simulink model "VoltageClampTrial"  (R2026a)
settings: Solver=ode1  StopTime=0.4  FixedStep=0.00001
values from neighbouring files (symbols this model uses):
  V_clamp = -0.065    [DataGeneration3.m]
libraries: LoomingNeuronLibrary x27

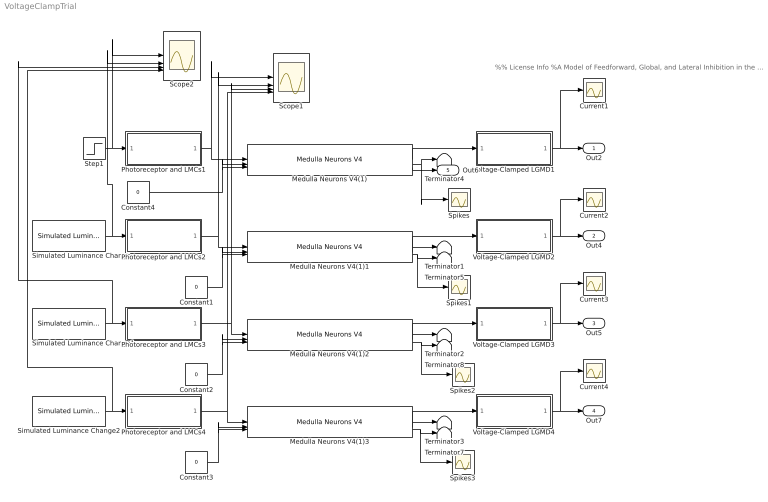
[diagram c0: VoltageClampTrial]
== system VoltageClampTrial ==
  note: %% License Info %A Model of Feedforward, Global, and Lateral Inhibition in the Locust Visual System. %This model examines the architecture and function of inhibitory mechanisms in the %visual system of locusts, namely those involved in the processing of inputs to a %key looming-sensitive neuron, the lobula giant movement detector (LGMD). %Copyright (c) 2026, Erik Olson, Travis Wiens, and Jack Gray %CITATION: %When using the model code for scientific publications, cite the following work: %Olson EGN, Wiens TK, Gray JR. A model of feedforward, global, and lateral inhibition %in the locust visual system predicts responses to looming stimuli. Biol Cybern. 2021 %Jun;115(3):245-265. doi: 10.1007/s00422-021-00876-8. Epub 2021 May 16. PMID: 33997912. %This program is free software: you can redistribute it and/or modify %it under the terms of the GNU General Public License as published by %the Free Software Foundation, either version 3 of the License, or %(at your option) any later version. %This program is distributed in the hope that it will be useful, %but WITHOUT ANY WARRANTY; without even the implied warranty of %MERCHANTABILITY or FITNESS FOR A PARTICULAR PURPOSE. See the %GNU General Public License for more details. %You should have received a copy of the GNU General Public License %along with this program. If not, see <https://www.gnu.org/licenses/>. %Contact: erik.olson@usask.ca
  Constant{1..4} (4 alike) : Constant  Value=0
  Current{1..4} (4 alike) : Scope
  Medulla Neurons V4(1){,1..3} (4 alike) : LoomingNeuronLibrary/Medulla Neurons V4  K_in_ex=K_E_m  K_in_lateral=0  K_in_global=0  g_m=g_L_m  c_m=c  E_rev_ex=E_E  E_rev_inh=E_I  E_rest=E_L  V_t=V_t  Delta_t=Delta_t_m  V_fire=V_fire  tau=tau_alpha_m  g_med_adap_inc=Delta_g_A_m  tau_med_adap=tau_A_m  E_rev_adap=E_A  g_noise=g_N_m  noise_T=T_noise  radius=1
  Photoreceptor and LMCs1 : Subsystem
  Photoreceptor and LMCs2 : Subsystem
  Photoreceptor and LMCs3 : Subsystem
  Photoreceptor and LMCs4 : Subsystem
  Scope1 : Scope  NumInputPorts=4
  Scope2 : Scope  NumInputPorts=4
  Simulated Luminance Change : LoomingNeuronLibrary/Simulated Luminance Change  duration=0.083  start=0
  Simulated Luminance Change1 : LoomingNeuronLibrary/Simulated Luminance Change  duration=0.183  start=0
  Simulated Luminance Change2 : LoomingNeuronLibrary/Simulated Luminance Change  duration=0.350  start=0
  Spikes{,1..3} (4 alike) : Scope
  Step1 : Step  Time=0.00001  InitialValue=1  FinalValue=0  SampleTime=0
  Terminator{1..5,7..8} (7 alike) : Terminator
  Voltage-Clamped LGMD1 : Subsystem
  Voltage-Clamped LGMD2 : Subsystem
  Voltage-Clamped LGMD3 : Subsystem
  Voltage-Clamped LGMD4 : Subsystem
  Out2 : Outport  VectorParamsAs1DForOutWhenUnconnected=off
  Out4 : Outport  Port=2  VectorParamsAs1DForOutWhenUnconnected=off
  Out5 : Outport  Port=3  VectorParamsAs1DForOutWhenUnconnected=off
  Out7 : Outport  Port=4  VectorParamsAs1DForOutWhenUnconnected=off
  Out6 : Outport  Port=5  VectorParamsAs1DForOutWhenUnconnected=off
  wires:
  Simulated Luminance Change/1 -> Photoreceptor and LMCs2/1(In1), Scope2/2
  Photoreceptor and LMCs4/1(Out1) -> Medulla Neurons V4(1)3/1, Scope1/4
  Medulla Neurons V4(1)2/1 -> Voltage-Clamped LGMD3/1(In1)
  Photoreceptor and LMCs2/1(Out1) -> Medulla Neurons V4(1)1/1, Scope1/2
  Simulated Luminance Change1/1 -> Photoreceptor and LMCs3/1(In1), Scope2/3
  Photoreceptor and LMCs1/1(Out1) -> Medulla Neurons V4(1)/1, Scope1/1
  Medulla Neurons V4(1)3/2 -> Terminator3/1
  Medulla Neurons V4(1)3/3 -> Spikes3/1, Terminator7/1
  Medulla Neurons V4(1)2/2 -> Terminator2/1
  Medulla Neurons V4(1)2/3 -> Spikes2/1, Terminator8/1
  Constant3/1 -> Medulla Neurons V4(1)3/3, Medulla Neurons V4(1)3/2
  Medulla Neurons V4(1)3/1 -> Voltage-Clamped LGMD4/1(In1)
  Voltage-Clamped LGMD4/1(Out1) -> Out7/1, Current4/1
  Medulla Neurons V4(1)1/2 -> Terminator1/1
  Medulla Neurons V4(1)1/3 -> Spikes1/1, Terminator5/1
  Photoreceptor and LMCs3/1(Out1) -> Medulla Neurons V4(1)2/1, Scope1/3
  Medulla Neurons V4(1)/1 -> Voltage-Clamped LGMD1/1(In1)
  Medulla Neurons V4(1)/3 -> Out6/1
  Step1/1 -> Scope2/1, Photoreceptor and LMCs1/1(In1)
  Voltage-Clamped LGMD3/1(Out1) -> Out5/1, Current3/1
  Medulla Neurons V4(1)/2 -> Spikes/1, Terminator4/1
  Medulla Neurons V4(1)1/1 -> Voltage-Clamped LGMD2/1(In1)
  Voltage-Clamped LGMD1/1(Out1) -> Out2/1, Current1/1
  Constant4/1 -> Medulla Neurons V4(1)/2, Medulla Neurons V4(1)/3
  Voltage-Clamped LGMD2/1(Out1) -> Out4/1, Current2/1
  Constant2/1 -> Medulla Neurons V4(1)2/2, Medulla Neurons V4(1)2/3
  Simulated Luminance Change2/1 -> Photoreceptor and LMCs4/1(In1), Scope2/4
  Constant1/1 -> Medulla Neurons V4(1)1/3, Medulla Neurons V4(1)1/2

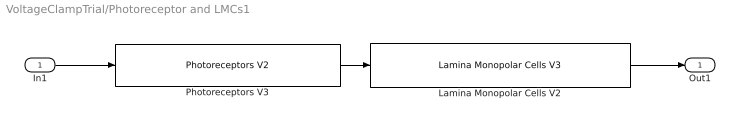
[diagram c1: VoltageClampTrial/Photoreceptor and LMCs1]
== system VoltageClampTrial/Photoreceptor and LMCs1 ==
  In1 : Inport
  Lamina Monopolar Cells V2 : LoomingNeuronLibrary/Lamina Monopolar Cells V3  K_LMC=K_LMC  gamma_1=b
  Photoreceptors V3 : LoomingNeuronLibrary/Photoreceptors V2  K_photoD=K_photoD  K_photoP=K_photoP  alpha_1=a_1  alpha_2=a_2
  Out1 : Outport  VectorParamsAs1DForOutWhenUnconnected=off
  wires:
  Lamina Monopolar Cells V2/1 -> Out1/1
  Photoreceptors V3/1 -> Lamina Monopolar Cells V2/1
  In1/1 -> Photoreceptors V3/1

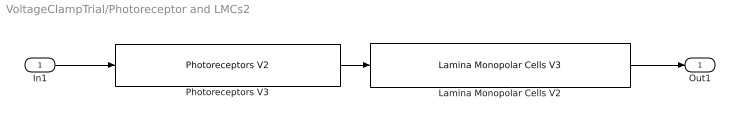
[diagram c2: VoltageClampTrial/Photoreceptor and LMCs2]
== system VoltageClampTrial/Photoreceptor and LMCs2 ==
  In1 : Inport
  Lamina Monopolar Cells V2 : LoomingNeuronLibrary/Lamina Monopolar Cells V3  K_LMC=K_LMC  gamma_1=b
  Photoreceptors V3 : LoomingNeuronLibrary/Photoreceptors V2  K_photoD=K_photoD  K_photoP=K_photoP  alpha_1=a_1  alpha_2=a_2
  Out1 : Outport  VectorParamsAs1DForOutWhenUnconnected=off
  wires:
  Lamina Monopolar Cells V2/1 -> Out1/1
  Photoreceptors V3/1 -> Lamina Monopolar Cells V2/1
  In1/1 -> Photoreceptors V3/1

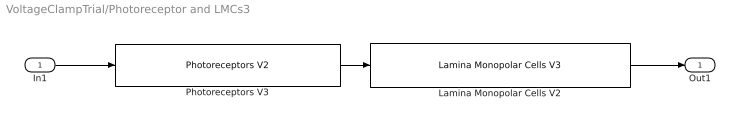
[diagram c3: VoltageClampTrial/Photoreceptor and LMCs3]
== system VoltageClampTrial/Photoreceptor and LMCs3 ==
  In1 : Inport
  Lamina Monopolar Cells V2 : LoomingNeuronLibrary/Lamina Monopolar Cells V3  K_LMC=K_LMC  gamma_1=b
  Photoreceptors V3 : LoomingNeuronLibrary/Photoreceptors V2  K_photoD=K_photoD  K_photoP=K_photoP  alpha_1=a_1  alpha_2=a_2
  Out1 : Outport  VectorParamsAs1DForOutWhenUnconnected=off
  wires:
  Lamina Monopolar Cells V2/1 -> Out1/1
  Photoreceptors V3/1 -> Lamina Monopolar Cells V2/1
  In1/1 -> Photoreceptors V3/1

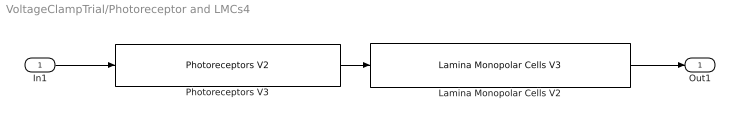
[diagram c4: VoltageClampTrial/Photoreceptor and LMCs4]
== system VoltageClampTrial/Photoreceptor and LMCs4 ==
  In1 : Inport
  Lamina Monopolar Cells V2 : LoomingNeuronLibrary/Lamina Monopolar Cells V3  K_LMC=K_LMC  gamma_1=b
  Photoreceptors V3 : LoomingNeuronLibrary/Photoreceptors V2  K_photoD=K_photoD  K_photoP=K_photoP  alpha_1=a_1  alpha_2=a_2
  Out1 : Outport  VectorParamsAs1DForOutWhenUnconnected=off
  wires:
  Lamina Monopolar Cells V2/1 -> Out1/1
  Photoreceptors V3/1 -> Lamina Monopolar Cells V2/1
  In1/1 -> Photoreceptors V3/1

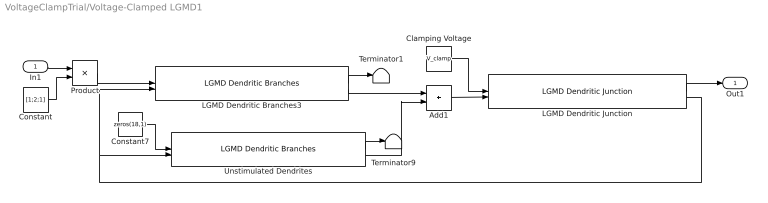
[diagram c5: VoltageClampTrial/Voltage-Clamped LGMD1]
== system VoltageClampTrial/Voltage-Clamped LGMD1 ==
  In1 : Inport
  Add1 : Sum
  Clamping Voltage : Constant  Value=V_clamp
  Constant : Constant  Value=[1;2;1]
  Constant7 : Constant  Value=zeros(18,1)
  LGMD Dendritic Branches3 : LoomingNeuronLibrary/LGMD Dendritic Branches  K_in=K_E_b  A_m=A_m_b  G_m=g_L_LGMD  G_b_j=G_b_j  C_m=c  E_rev=E_E  E_rest=E_L
  LGMD Dendritic Junction : LoomingNeuronLibrary/LGMD Dendritic Junction  A_m=A_m_j  G_j_c=G_j_c  G_m=g_L_LGMD  C_m=c  E_rest=E_L
  Product : Product
  Terminator1 : Terminator
  Terminator9 : Terminator
  Unstimulated Dendrites : LoomingNeuronLibrary/LGMD Dendritic Branches  K_in=K_E_b  A_m=A_m_b  G_m=g_L_LGMD  G_b_j=G_b_j  C_m=c  E_rev=E_E  E_rest=E_L
  Out1 : Outport  VectorParamsAs1DForOutWhenUnconnected=off
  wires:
  LGMD Dendritic Junction/2 -> LGMD Dendritic Branches3/2, Unstimulated Dendrites/2
  LGMD Dendritic Junction/1 -> Out1/1
  Add1/1 -> LGMD Dendritic Junction/2
  Clamping Voltage/1 -> LGMD Dendritic Junction/1
  Unstimulated Dendrites/2 -> Add1/2
  LGMD Dendritic Branches3/1 -> Terminator1/1
  Unstimulated Dendrites/1 -> Terminator9/1
  LGMD Dendritic Branches3/2 -> Add1/1
  Constant7/1 -> Unstimulated Dendrites/1
  Product/1 -> LGMD Dendritic Branches3/1
  In1/1 -> Product/1
  Constant/1 -> Product/2

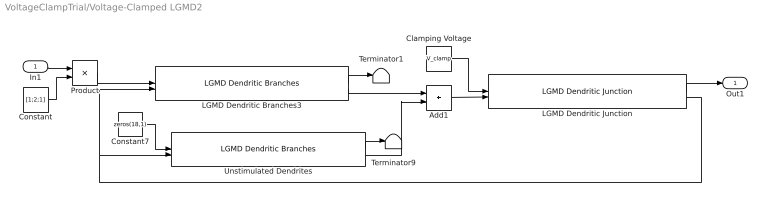
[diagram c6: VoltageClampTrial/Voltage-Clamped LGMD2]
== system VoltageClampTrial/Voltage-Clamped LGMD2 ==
  In1 : Inport
  Add1 : Sum
  Clamping Voltage : Constant  Value=V_clamp
  Constant : Constant  Value=[1;2;1]
  Constant7 : Constant  Value=zeros(18,1)
  LGMD Dendritic Branches3 : LoomingNeuronLibrary/LGMD Dendritic Branches  K_in=K_E_b  A_m=A_m_b  G_m=g_L_LGMD  G_b_j=G_b_j  C_m=c  E_rev=E_E  E_rest=E_L
  LGMD Dendritic Junction : LoomingNeuronLibrary/LGMD Dendritic Junction  A_m=A_m_j  G_j_c=G_j_c  G_m=g_L_LGMD  C_m=c  E_rest=E_L
  Product : Product
  Terminator1 : Terminator
  Terminator9 : Terminator
  Unstimulated Dendrites : LoomingNeuronLibrary/LGMD Dendritic Branches  K_in=K_E_b  A_m=A_m_b  G_m=g_L_LGMD  G_b_j=G_b_j  C_m=c  E_rev=E_E  E_rest=E_L
  Out1 : Outport  VectorParamsAs1DForOutWhenUnconnected=off
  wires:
  LGMD Dendritic Junction/2 -> LGMD Dendritic Branches3/2, Unstimulated Dendrites/2
  LGMD Dendritic Junction/1 -> Out1/1
  Add1/1 -> LGMD Dendritic Junction/2
  Clamping Voltage/1 -> LGMD Dendritic Junction/1
  Unstimulated Dendrites/2 -> Add1/2
  LGMD Dendritic Branches3/1 -> Terminator1/1
  Unstimulated Dendrites/1 -> Terminator9/1
  LGMD Dendritic Branches3/2 -> Add1/1
  Constant7/1 -> Unstimulated Dendrites/1
  Product/1 -> LGMD Dendritic Branches3/1
  In1/1 -> Product/1
  Constant/1 -> Product/2

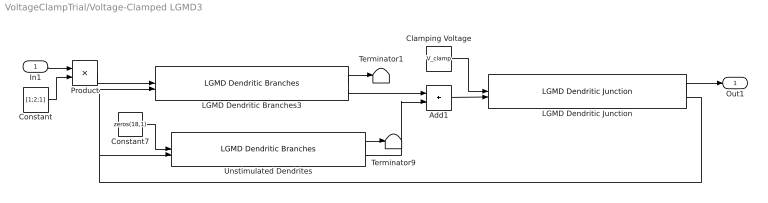
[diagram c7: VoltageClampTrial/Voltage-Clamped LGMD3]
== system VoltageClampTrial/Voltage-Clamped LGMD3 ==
  In1 : Inport
  Add1 : Sum
  Clamping Voltage : Constant  Value=V_clamp
  Constant : Constant  Value=[1;2;1]
  Constant7 : Constant  Value=zeros(18,1)
  LGMD Dendritic Branches3 : LoomingNeuronLibrary/LGMD Dendritic Branches  K_in=K_E_b  A_m=A_m_b  G_m=g_L_LGMD  G_b_j=G_b_j  C_m=c  E_rev=E_E  E_rest=E_L
  LGMD Dendritic Junction : LoomingNeuronLibrary/LGMD Dendritic Junction  A_m=A_m_j  G_j_c=G_j_c  G_m=g_L_LGMD  C_m=c  E_rest=E_L
  Product : Product
  Terminator1 : Terminator
  Terminator9 : Terminator
  Unstimulated Dendrites : LoomingNeuronLibrary/LGMD Dendritic Branches  K_in=K_E_b  A_m=A_m_b  G_m=g_L_LGMD  G_b_j=G_b_j  C_m=c  E_rev=E_E  E_rest=E_L
  Out1 : Outport  VectorParamsAs1DForOutWhenUnconnected=off
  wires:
  LGMD Dendritic Junction/2 -> LGMD Dendritic Branches3/2, Unstimulated Dendrites/2
  LGMD Dendritic Junction/1 -> Out1/1
  Add1/1 -> LGMD Dendritic Junction/2
  Clamping Voltage/1 -> LGMD Dendritic Junction/1
  Unstimulated Dendrites/2 -> Add1/2
  LGMD Dendritic Branches3/1 -> Terminator1/1
  Unstimulated Dendrites/1 -> Terminator9/1
  LGMD Dendritic Branches3/2 -> Add1/1
  Constant7/1 -> Unstimulated Dendrites/1
  Product/1 -> LGMD Dendritic Branches3/1
  In1/1 -> Product/1
  Constant/1 -> Product/2

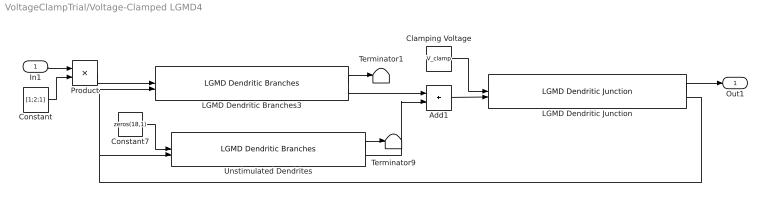
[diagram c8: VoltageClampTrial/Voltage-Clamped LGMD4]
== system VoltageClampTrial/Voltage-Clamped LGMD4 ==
  In1 : Inport
  Add1 : Sum
  Clamping Voltage : Constant  Value=V_clamp
  Constant : Constant  Value=[1;2;1]
  Constant7 : Constant  Value=zeros(18,1)
  LGMD Dendritic Branches3 : LoomingNeuronLibrary/LGMD Dendritic Branches  K_in=K_E_b  A_m=A_m_b  G_m=g_L_LGMD  G_b_j=G_b_j  C_m=c  E_rev=E_E  E_rest=E_L
  LGMD Dendritic Junction : LoomingNeuronLibrary/LGMD Dendritic Junction  A_m=A_m_j  G_j_c=G_j_c  G_m=g_L_LGMD  C_m=c  E_rest=E_L
  Product : Product
  Terminator1 : Terminator
  Terminator9 : Terminator
  Unstimulated Dendrites : LoomingNeuronLibrary/LGMD Dendritic Branches  K_in=K_E_b  A_m=A_m_b  G_m=g_L_LGMD  G_b_j=G_b_j  C_m=c  E_rev=E_E  E_rest=E_L
  Out1 : Outport  VectorParamsAs1DForOutWhenUnconnected=off
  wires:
  LGMD Dendritic Junction/2 -> LGMD Dendritic Branches3/2, Unstimulated Dendrites/2
  LGMD Dendritic Junction/1 -> Out1/1
  Add1/1 -> LGMD Dendritic Junction/2
  Clamping Voltage/1 -> LGMD Dendritic Junction/1
  Unstimulated Dendrites/2 -> Add1/2
  LGMD Dendritic Branches3/1 -> Terminator1/1
  Unstimulated Dendrites/1 -> Terminator9/1
  LGMD Dendritic Branches3/2 -> Add1/1
  Constant7/1 -> Unstimulated Dendrites/1
  Product/1 -> LGMD Dendritic Branches3/1
  In1/1 -> Product/1
  Constant/1 -> Product/2
